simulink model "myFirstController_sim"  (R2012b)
settings: Solver=ode45  StartTime=0.0  StopTime=60  RelTol=1e-3
PreLoadFcn:
  | load myFirstController_data.mat
InitFcn:
  | configure_block
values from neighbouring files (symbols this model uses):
  A = [0.7115 -0.4345; 0.4345 0.8853]    [simCLoop.m]    (also in myforcespro.m = [   0.7115  -0.4345;          0.4345  0.8853  ])
  B = [0.2173;0.0573]    [simCLoop.m]    (also in myforcespro.m = [   0.2173;          0.0573  ])
  C = [0 1]    [simCLoop.m]

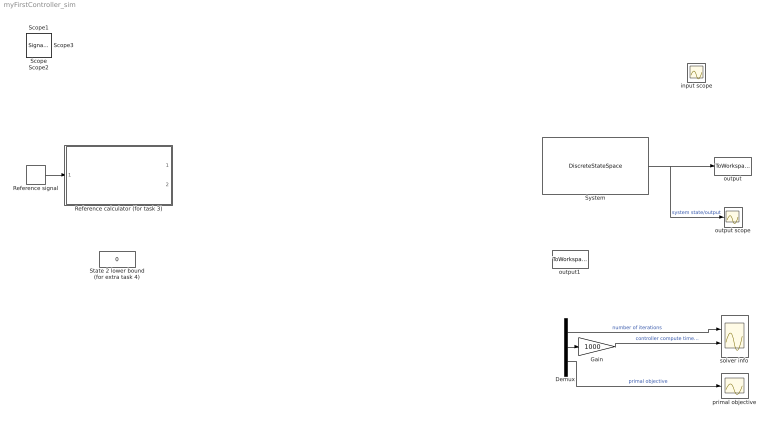
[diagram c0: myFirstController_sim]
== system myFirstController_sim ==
  Demux : Demux  Outputs=3
  Gain : Gain  Gain=1000
  Reference calculator (for task 3) : Subsystem
  Reference signal : DiscretePulseGenerator  PulseType=Time based  Amplitude=2  Period=40  PulseWidth=50  PhaseDelay=5
  State 2 lower bound (for extra task 4) : Constant  Value=0
  System : DiscreteStateSpace  A=A  B=B  C=C  D=zeros(2,1)  X0=[0; 6]
  input scope : Scope
  output : ToWorkspace  VariableName=simulink_res  SampleTime=-1  SaveFormat=Timeseries
  output scope : Scope
  output1 : ToWorkspace  VariableName=solverinfo  SampleTime=-1  SaveFormat=Timeseries
  primal objective : Scope
  solver info : Scope  NumInputPorts=2
  Scope : SignalViewerScope  IOType=viewer  ZoomMode=yonly  RefreshTime=0.035000
  Scope1 : SignalViewerScope  IOType=viewer  RefreshTime=0.035000
  Scope2 : SignalViewerScope  IOType=viewer  RefreshTime=0.035000
  Scope3 : SignalViewerScope  IOType=viewer  RefreshTime=0.035000
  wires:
  System/1 -> output/1, output scope/1  "system state/output"
  ? -> Demux/1, output1/1  "solver info"
  Demux/2 -> Gain/1
  Gain/1 -> solver info/2  "controller compute time in ms"
  Demux/1 -> solver info/1  "number of iterations"
  Demux/3 -> primal objective/1  "primal objective"
  Reference signal/1 -> Reference calculator (for task 3)/1(Output reference)
  ? -> input scope/1, System/1

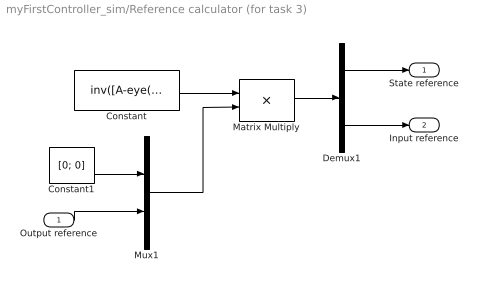
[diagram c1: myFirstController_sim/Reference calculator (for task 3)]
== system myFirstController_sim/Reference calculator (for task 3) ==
  Output reference : Inport
  Constant : Constant  Value=inv([A-eye(2), B; 0 1 0])
  Constant1 : Constant  Value=[0; 0]
  Demux1 : Demux  Outputs=[2 1]
  Matrix Multiply : Product  Multiplication=Matrix(*)
  Mux1 : Mux  Inputs=2
  State reference : Outport
  Input reference : Outport  Port=2
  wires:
  Mux1/1 -> Matrix Multiply/2
  Demux1/2 -> Input reference/1
  Matrix Multiply/1 -> Demux1/1
  Constant1/1 -> Mux1/1
  Demux1/1 -> State reference/1
  Output reference/1 -> Mux1/2
  Constant/1 -> Matrix Multiply/1
